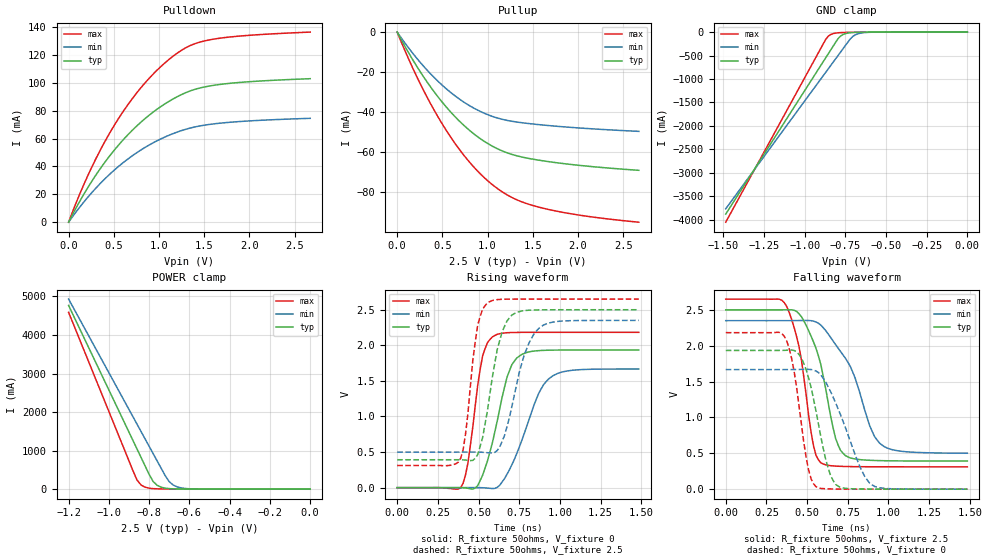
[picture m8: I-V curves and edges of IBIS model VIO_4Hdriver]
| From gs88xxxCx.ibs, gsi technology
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|  signals   DQA1-DQA9, DQB1-DQB9, DQC1-DQC9, DQD1-DQD9
[Model]   VIO_4Hdriver
Model_type   I/O
Polarity   Non-Inverting
Vinl  =   0.54v
Vinh  =   1.10v
Vmeas =   0.90v
Cref  =   0pF
Rref  =   50
Vref  =   0.90v
|  variable   typ   min   max
C_comp   3.0pF   2.5pF   3.5pF
|  variable   typ   min   max
[Temperature Range]   50   0   100
|  variable   typ   min   max
[Voltage Range]   2.5   2.35   2.65
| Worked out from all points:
|   slope of the pulldown table from 0 to 0.375 V, typ, clamps not added: 9.23 ohm
|   slope of the pullup table from 0 to 0.375 V, typ, clamps not added: 13.5 ohm
|   GND clamp passes 1 mA (typ) near -0.61 V on its own axis
|   POWER clamp passes 1 mA (typ) near -0.59 V on its own axis
|   rising waveform, R_fixture 50ohms, V_fixture 0: 20-80 % time 118ps typ, 165ps min, 76.5ps max; typ from 0 V to 1.93 V
|   rising waveform, R_fixture 50ohms, V_fixture 2.5: 20-80 % time 97.7ps typ, 125ps min, 66.9ps max; typ from 0.392 V to 2.5 V
|   falling waveform, R_fixture 50ohms, V_fixture 2.5: 20-80 % time 129ps typ, 201ps min, 96.6ps max; typ from 2.5 V to 0.392 V
|   falling waveform, R_fixture 50ohms, V_fixture 0: 20-80 % time 108ps typ, 171ps min, 83.2ps max; typ from 1.93 V to 0 V
[Pulldown]
| voltage   typ   min   max
0V        -364.2pA   -1.049nA   -219.7pA
108mV     13.2mA     9.526mA    17.82mA
243mV     27.94mA    20.19mA    37.64mA
378mV     40.9mA     29.57mA    55.04mA
513mV     52.26mA    37.78mA    70.27mA
648mV     62.15mA    44.92mA    83.54mA
810mV     72.28mA    52.18mA    97.18mA
1.134V    87.55mA    62.95mA    117.9mA
1.35V     94.22mA    67.56mA    126.7mA
1.566V    97.72mA    70.15mA    130.8mA
1.971V    100.6mA    72.49mA    133.8mA
2.673V    102.9mA    74.48mA    136.3mA
[Pullup]
| voltage (VDDQ-Vout)   typ   min   max
0V        266.7pA    1.042nA    119pA
243mV     -19.01mA   -14.52mA   -24.74mA
378mV     -27.99mA   -21.3mA    -36.57mA
513mV     -35.9mA    -27.19mA   -47.06mA
648mV     -42.73mA   -32.2mA    -56.26mA
783mV     -48.53mA   -36.37mA   -64.19mA
918mV     -53.32mA   -39.7mA    -70.9mA
1.053V    -57.13mA   -42.21mA   -76.41mA
1.296V    -61.61mA   -44.86mA   -83.41mA
1.566V    -64.13mA   -46.34mA   -87.65mA
2.025V    -66.79mA   -48.05mA   -91.73mA
2.673V    -69.22mA   -49.72mA   -95.2mA
[GND Clamp]
| voltage   typ   min   max
-1.485V   -3.884A    -3.771A    -4.056A
-885mV    -626.9mA   -926.9mA   -247.2mA
-870mV    -545.6mA   -856mA     -153.5mA
-855mV    -464.4mA   -785mA     -89.11mA
-825mV    -301.9mA   -643.2mA   -32.88mA
-795mV    -141.5mA   -501.4mA   -15.38mA
-780mV    -86.61mA   -430.5mA   -11.65mA
-750mV    -32.85mA   -288.8mA   -7.734mA
-705mV    -8.727mA   -95.28mA   -4.834mA
-660mV    -2.907mA   -24.97mA   -2.925mA
-555mV    -316.7uA   -1.176mA   -484.9uA
0V        -354.4pA   -1.034nA   -211.5pA
[POWER Clamp]
| voltage (VDDQ-Vout)   typ   min   max
-1.2V     4.765A     4.931A     4.585A
-880mV    1.258A     1.875A     474.1mA
-860mV    1.039A     1.684A     234.3mA
-840mV    820.4mA    1.493A     107.4mA
-820mV    601.5mA    1.302A     50.64mA
-780mV    197.3mA    920.5mA    14.28mA
-760mV    99.71mA    729.7mA    9.034mA
-720mV    26.23mA    348.2mA    4.898mA
-700mV    13.96mA    192.6mA    3.916mA
-660mV    4.495mA    57.55mA    2.579mA
-560mV    510.5uA    2.941mA    648.3uA
0V        285pA      1.042nA    119.1pA
[Ramp]
| voltage   typ   min   max
dV/dt_r   0.73/293p   0.46/457p   0.95/179p
dV/dt_f   0.76/309p   0.57/651p   0.94/178p
R_load  =   50ohms
[Rising Waveform]
C_fixture =   0.0pF
R_fixture =   50ohms
V_fixture =   0
| Time   V(typ)   V(min)   V(max)
0s        2.453nV    9.321nV    1.135nV
390ps     -117.1uV   269.4uV    -1.014mV
435ps     -9.102mV   542.7uV    347.2mV
525ps     173.6mV    -1.26mV    1.849V
585ps     628.1mV    -12.57mV   2.118V
675ps     1.553V     188.7mV    2.177V
765ps     1.871V     658.5mV    2.182V
870ps     1.925V     1.326V     2.183V
960ps     1.933V     1.576V     2.183V
1.485ns   1.934V     1.667V     2.183V
[Rising Waveform]
C_fixture =   0.0pF
R_fixture =   50ohms
V_fixture =   2.5
V_fixture_min =  2.35
V_fixture_max =  2.65
| Time   V(typ)   V(min)   V(max)
0s        392.1mV    499.5mV    311.6mV
390ps     391.5mV    499.8mV    411.9mV
420ps     387.8mV    500mV      749.7mV
495ps     465.6mV    499.2mV    2.285V
555ps     1.085V     490.9mV    2.598V
615ps     1.94V      522.7mV    2.642V
675ps     2.343V     858mV      2.648V
780ps     2.486V     1.859V     2.65V
870ps     2.498V     2.238V     2.65V
1.485ns   2.5V       2.35V      2.65V
[Falling Waveform]
C_fixture =   0.0pF
R_fixture =   50ohms
V_fixture =   2.5
V_fixture_min =  2.35
V_fixture_max =  2.65
| Time   V(typ)   V(min)   V(max)
0s        2.5V       2.35V      2.65V
375ps     2.501V     2.35V      2.546V
465ps     2.406V     2.352V     1.805V
540ps     2.05V      2.342V     599.5mV
585ps     1.732V     2.286V     366.7mV
675ps     710.4mV    2.016V     321.8mV
735ps     468.9mV    1.827V     316.4mV
885ps     402.7mV    883.2mV    312.5mV
945ps     398.1mV    642.8mV    312mV
1.485ns   392.2mV    501.2mV    311.6mV
[Falling Waveform]
C_fixture =   0.0pF
R_fixture =   50ohms
V_fixture =   0
| Time   V(typ)   V(min)   V(max)
0s        1.934V     1.667V     2.183V
360ps     1.936V     1.667V     2.131V
405ps     1.94V      1.668V     1.823V
465ps     1.829V     1.67V      908mV
510ps     1.544V     1.67V      262.6mV
555ps     1.088V     1.647V     32.71mV
615ps     409.5mV    1.491V     5.505mV
675ps     67.11mV    1.206V     1.955mV
885ps     1.273mV    82.85mV    159.1uV
1.485ns   6.403uV    99.65uV    776nV
